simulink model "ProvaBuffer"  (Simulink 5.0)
settings: Solver=ode45  StartTime=0.0  StopTime=8  RelTol=1e-3

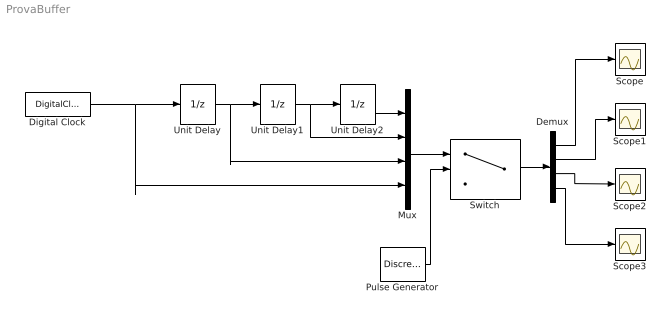
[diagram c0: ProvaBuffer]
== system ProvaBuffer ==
  Demux : Demux
  Digital Clock : DigitalClock
  Mux : Mux
  Pulse Generator : DiscretePulseGenerator  PulseType=Time based  Period=4  PulseWidth=0.1
  Scope{,1..3} (4 alike) : Scope
  Switch : Switch  Threshold=1
  Unit Delay : UnitDelay
  Unit Delay1 : UnitDelay
  Unit Delay2 : UnitDelay
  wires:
  Unit Delay/1 -> Unit Delay1/1, Mux/3
  Unit Delay1/1 -> Unit Delay2/1, Mux/2
  Digital Clock/1 -> Unit Delay/1, Mux/4
  Unit Delay2/1 -> Mux/1
  Mux/1 -> Switch/1
  Pulse Generator/1 -> Switch/2
  Switch/1 -> Demux/1
  Demux/1 -> Scope/1
  Demux/2 -> Scope1/1
  Demux/3 -> Scope2/1
  Demux/4 -> Scope3/1
